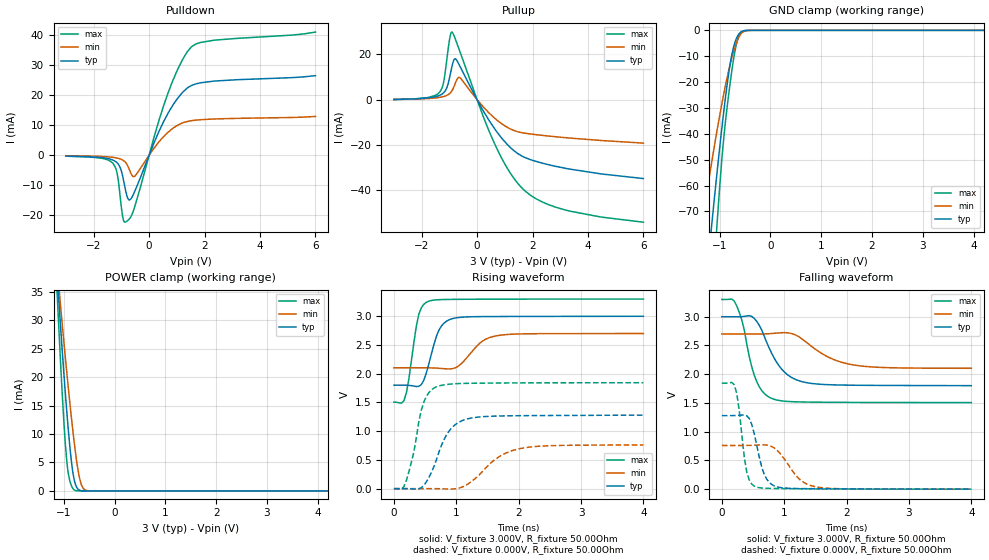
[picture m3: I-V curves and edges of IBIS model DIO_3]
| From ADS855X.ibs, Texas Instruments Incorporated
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|   I/O 3.0V Model
[Model]   DIO_3
Model_type   I/O
|Polarity   Non-Inverting
Enable   Active-High
|Signals   DB14/REFBUFEN, DB13/SDI, DB12, DB11, DB10/SDO_C, DB9/SDO_B
|   DB8/SDO_A, DB7/HBEN/DCEN, DB6/SCLK, DB5/DCIN_A, DB4/DCIN_B,
|   DB3/DCIN_C, DB2/SEL_C, DB1/SEL_B, DB0/SEL_A, RANGE/XCLK,
|   DB15
Vinl = -300.000mV   |min, BGND -0.3V
Vinh = 3.6V   |max. BVDD +0.3V
Vmeas = 1.496V
Cref = 30.00pF
Rref = 82   |For BVDD=2.7 [{0.3*BVDD/Imax}-Rout(max) with Imax=5mA, Rout_max=80ohm]
| C_comp   obtained at 25MHz
| variable   typ   min   max
|C_comp Output Disable
C_comp   3.773pF   2.857pF   4.603pF
|C_comp Output Low
|C_comp   4.145pF   3.198pF   4.983pF
|C_comp Output High
|C_comp   4.213pF   3.266pF   5.127pF
[Model Spec]
|Timing spec test load voltage corners 0.5*VCC
Vmeas   1.50V   1.34V   1.74V
Vref   2.50V   0.50V   3.00V
|Junction Temperature
[Temperature Range]   40.0   125.0   -40.0
[Voltage range]   3.0V   2.7V   3.3V
[Pullup reference]   3.0V   2.7V   3.3V
[power clamp reference]   3.0V   2.7V   3.3V
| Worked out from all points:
|   slope of the pulldown table from 0 to 0.45 V, typ, clamps not added: 46 ohm
|   slope of the pullup table from 0 to 0.45 V, typ, clamps not added: 47.3 ohm
|   GND clamp passes 1 mA (typ) near -0.60 V on its own axis
|   POWER clamp passes 1 mA (typ) near -0.76 V on its own axis
|   falling waveform, V_fixture 3.000V, R_fixture 50.00Ohm: 20-80 % time 358ps typ, 551ps min, 241ps max; typ from 3 V to 1.8 V
|   rising waveform, V_fixture 3.000V, R_fixture 50.00Ohm: 20-80 % time 196ps typ, 315ps min, 149ps max; typ from 1.8 V to 3 V
|   rising waveform, V_fixture 0.000V, R_fixture 50.00Ohm: 20-80 % time 312ps typ, 498ps min, 212ps max; typ from 0 V to 1.28 V
|   falling waveform, V_fixture 0.000V, R_fixture 50.00Ohm: 20-80 % time 176ps typ, 326ps min, 124ps max; typ from 1.28 V to 0 V
[Pulldown]
|   Voltage   I(typ)   I(min)   I(max)
-3V       -311.4uA   -196.7uA   -346.8uA
-1.308V   -1.633mA   -731.7uA   -2.699mA
-1.154V   -2.588mA   -968.7uA   -6.156mA
-1.028V   -4.599mA   -1.309mA   -15.32mA
-939mV    -7.716mA   -1.721mA   -21.19mA
-852.4mV  -11.65mA   -2.418mA   -22.27mA
-715.1mV  -14.91mA   -4.76mA    -21.23mA
-539.6mV  -12.46mA   -7.12mA    -17.68mA
620.2mV   12.92mA    7.091mA    19.09mA
1.039V    19.07mA    10.02mA    28.74mA
1.52V     23.15mA    11.46mA    35.99mA
5.999V    26.47mA    12.88mA    40.98mA
[GND Clamp]
|   Voltage   I(typ)   I(min)   I(max)
-3V       -493.1mA   -328.5mA   -702.2mA
-1.383V   -122.5mA   -79.89mA   -177.4mA
-1.326V   -110.4mA   -72.39mA   -159.3mA
-1.179V   -80.14mA   -53.91mA   -113.4mA
-1.121V   -68.8mA    -47.05mA   -96.04mA
-1.054V   -55.86mA   -39.26mA   -76.29mA
-917.6mV  -31.58mA   -24.69mA   -41.86mA
-787.1mV  -12.59mA   -12.82mA   -19.83mA
-721.9mV  -6.351mA   -8.03mA    -10.97mA
-660mV    -2.796mA   -4.418mA   -4.757mA
-549.8mV  -340.5uA   -799.5uA   -408.9uA
5.999V    42.07nA    54.01nA    30.24nA
[Pullup]
|   Voltage   I(typ)   I(min)   I(max)
-3V       89.08uA    84.11uA    67.2uA
-1.352V   1.893mA    1.002mA    3.327mA
-1.206V   3.068mA    1.385mA    7.796mA
-996.4mV  9.512mA    2.653mA    26.38mA
-910.9mV  14.45mA    3.885mA    29.91mA
-792.8mV  18.13mA    7.063mA    27.08mA
-612.8mV  14.64mA    9.666mA    21.08mA
664.1mV   -13.42mA   -8.5mA     -20.34mA
1.146V    -20.51mA   -12.59mA   -31.46mA
1.644V    -25.14mA   -14.68mA   -39.42mA
3.226V    -30.47mA   -16.87mA   -48.97mA
5.999V    -34.92mA   -19.23mA   -54.23mA
[POWER Clamp]
|   Voltage   I(typ)   I(min)   I(max)
-3V       226.3mA    192mA      270.5mA
-1.136V   38.85mA    40.03mA    35.99mA
-1.107V   34.88mA    37.04mA    30.59mA
-1.072V   30.23mA    33.52mA    24.33mA
-996.4mV  20.62mA    26.16mA    12.09mA
-939mV    13.94mA    20.82mA    5.225mA
-910.9mV  10.94mA    18.28mA    3.164mA
-845.6mV  5.024mA    12.67mA    875.5uA
-773.6mV  1.289mA    7.125mA    95.94uA
-656.6mV  44.02uA    1.217mA    1.965uA
-494.6mV  190nA      16.18uA    23.79nA
5.999V    -35.58nA   -43.76nA   -27.45nA
[Ramp]
R_load = 50.00Ohm
|   typ   min   max
dV/dt_r   767.588mV/312.053ps 456.037mV/498.259ps   1.106V/212.284ps
dV/dt_f   719.581mV/357.804ps 358.322mV/551.033ps   1.076V/241.495ps
[Falling Waveform]
V_fixture = 3.000V
V_fixture_min = 2.700V
V_fixture_max = 3.300V
R_fixture = 50.00Ohm
|   Time   V(typ)   V(min)   V(max)
0s        3V         2.7V       3.3V
240ps     2.999V     2.7V       3.185V
320ps     3.001V     2.7V       2.942V
520ps     2.969V     2.699V     1.982V
640ps     2.768V     2.7V       1.716V
800ps     2.361V     2.708V     1.578V
1.04ns    2.002V     2.721V     1.527V
1.4ns     1.845V     2.517V     1.515V
2.16ns    1.808V     2.153V     1.509V
4ns       1.801V     2.103V     1.507V
[Rising Waveform]
V_fixture = 3.000V
V_fixture_min = 2.700V
V_fixture_max = 3.300V
R_fixture = 50.00Ohm
|   Time   V(typ)   V(min)   V(max)
0s        1.801V     2.103V     1.507V
160ps     1.801V     2.103V     1.53V
240ps     1.798V     2.103V     1.91V
400ps     1.78V      2.103V     3.039V
560ps     2.172V     2.103V     3.263V
720ps     2.755V     2.095V     3.289V
960ps     2.965V     2.094V     3.295V
1.4ns     2.994V     2.552V     3.297V
1.64ns    2.996V     2.66V      3.298V
4ns       3V         2.7V       3.3V
[Rising Waveform]
V_fixture = 0.000V
V_fixture_min = 0.000V
V_fixture_max = 0.000V
R_fixture = 50.00Ohm
|   Time   V(typ)   V(min)   V(max)
0s        -885.7nV   -1.489uV   -525.3nV
160ps     402.9uV    12.28uV    36.12mV
320ps     -6.54mV    181.6uV    640.9mV
480ps     56.13mV    449.8uV    1.508V
680ps     497.4mV    -760.7uV   1.771V
880ps     995mV      -6.603mV   1.817V
1.2ns     1.219V     89.7mV     1.833V
1.64ns    1.263V     520.9mV    1.838V
2ns       1.269V     691.2mV    1.84V
4ns       1.279V     760.1mV    1.844V
[Falling Waveform]
V_fixture = 0.000V
V_fixture_min = 0.000V
V_fixture_max = 0.000V
R_fixture = 50.00Ohm
|   Time   V(typ)   V(min)   V(max)
0s        1.279V     760.1mV    1.844V
200ps     1.28V      759.7mV    1.814V
280ps     1.285V     759.7mV    1.362V
400ps     1.277V     760.7mV    293.4mV
520ps     963.4mV    764.7mV    52.74mV
680ps     258mV      770.9mV    16.78mV
880ps     41.6mV     681.3mV    11.34mV
1.24ns    10.37mV    177.9mV    7.383mV
1.52ns    7.792mV    38.03mV    4.654mV
4ns       -885.7nV   -1.489uV   -525.3nV
